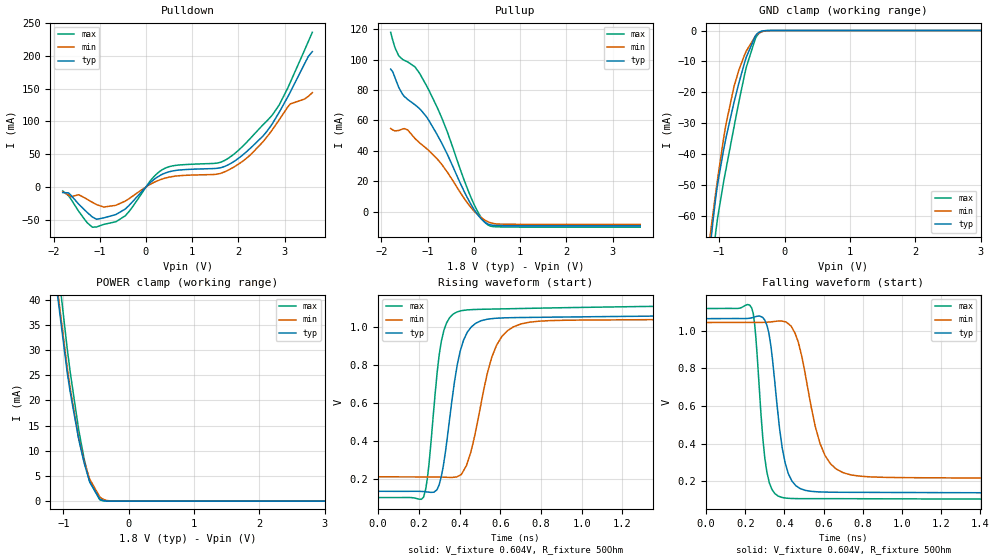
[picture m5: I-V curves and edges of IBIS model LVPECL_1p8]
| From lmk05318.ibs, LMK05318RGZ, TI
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|   LVPECL_1p8 Model
[Model]   LVPECL_1p8
Model_type   3-state
Polarity   Non-Inverting
Vmeas = 0.604
Vref = 0.604
Cref = 2pF
Rref = 50
|   typ   min   max
C_comp   1.5263E-12   1.43105E-12   1.63546E-12
| Where nom  PVT is Nominal Process, 1.8V, 27C
|   Fast PVT is Strong Process,  1.9V, -40C
|   Slow PVT is Weak Process,   1.7V, 125C
[Voltage Range]   1.8   1.7   1.9
|Junction Temperature
[Temperature Range]   27   125   -40
[Pullup Reference]   1.8   1.7   1.9
[Pulldown Reference]   -0   -0   0
[Power Clamp Reference]   1.8   1.7   1.9
[GND Clamp Reference]   0   0   0
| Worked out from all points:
|   slope of the pulldown table from 0 to 0.27 V, typ, clamps not added: 16.8 ohm
|   slope of the pullup table from 0 to 0.27 V, typ, clamps not added: 29.3 ohm
|   GND clamp passes 1 mA (typ) near -0.42 V on its own axis
|   POWER clamp passes 1 mA (typ) near -0.47 V on its own axis
|   falling waveform, V_fixture 0.604V, R_fixture 50Ohm: 20-80 % time 63.4ps typ, 105ps min, 44.6ps max; typ from 1.06 V to 0.136 V
|   rising waveform, V_fixture 0.604V, R_fixture 50Ohm: 20-80 % time 77.1ps typ, 108ps min, 56.9ps max; typ from 0.136 V to 1.06 V
[Pulldown]
|   Voltage   I(typ)   I(min)   I(max)
-1.8V     -8.523mA   -7.443mA   -6.058mA
-1.665V   -9.59mA    -12.82mA   -14.31mA
-1.271V   -38.91mA   -18.85mA   -54.56mA
-1.071V   -49.24mA   -26.78mA   -61.08mA
-444.6mV  -33.56mA   -21.46mA   -43.87mA
106.2mV   7.449mA    4.544mA    10.42mA
408.6mV   21.01mA    13.34mA    28.45mA
1.786V    33.99mA    25.83mA    43.93mA
2.531V    77.56mA    68.77mA    94.79mA
2.887V    114.4mA    102.9mA    125.6mA
3.125V    144.9mA    126.8mA    159.9mA
3.6V      206.5mA    143.9mA    236mA
[GND Clamp]
|   Voltage   I(typ)   I(min)   I(max)
-1.8V     -227.5mA   -244.3mA   -293.8mA
-1.125V   -67.81mA   -64.27mA   -79.09mA
-1.114V   -65.59mA   -62.48mA   -76.82mA
-1.093V   -61.33mA   -58.94mA   -72.53mA
-1.049V   -53.68mA   -52.02mA   -64.8mA
-909mV    -36.18mA   -32mA      -46.42mA
-768.6mV  -22.88mA   -17.82mA   -30.77mA
-585mV    -8.613mA   -6.634mA   -11.87mA
-444.6mV  -1.694mA   -1.777mA   -2.489mA
-385.2mV  -510.7uA   -772.5uA   -830.7uA
-217.8mV  -3.668uA   -26.55uA   -3.583uA
3.6V      0A         0A         0A
[Pullup]
|   Voltage   I(typ)   I(min)   I(max)
-1.8V     93.82mA    54.75mA    118.1mA
-1.708V   88.37mA    53.19mA    108.2mA
-1.627V   81.94mA    53.39mA    102.7mA
-1.433V   73.89mA    53.78mA    98.59mA
-1.265V   70.12mA    47.86mA    94.92mA
-973.8mV  60.02mA    40.15mA    79.97mA
-574.2mV  37.69mA    25.95mA    52.48mA
-72mV     5.208mA    2.981mA    9.959mA
90mV      -2.385mA   -2.254mA   -490uA
262.8mV   -7.547mA   -6.079mA   -7.877mA
522mV     -9.257mA   -8.251mA   -10.13mA
3.6V      -9.435mA   -8.467mA   -10.31mA
[POWER Clamp]
|   Voltage   I(typ)   I(min)   I(max)
-1.8V     167.1mA    290.8mA    175.6mA
-1.103V   42.32mA    43.41mA    48.96mA
-941.4mV  25.56mA    26.6mA     30.29mA
-892.8mV  21.47mA    22.2mA     25.41mA
-774mV    12.9mA     13.11mA    14.91mA
-752.4mV  11.54mA    11.74mA    13.24mA
-682.2mV  7.588mA    7.904mA    8.398mA
-595.8mV  3.783mA    4.344mA    3.83mA
-444.6mV  459.2uA    875.5uA    303.4uA
-352.8mV  57.32uA    198.5uA    23.38uA
-201.6mV  542.8nA    8.178uA    29.43nA
3.6V      0A         0A         0A
[Ramp]
R_load = 50
|   typ   min   max
dV/dt_r   0.557134/7.71003e-11   0.499157/1.08189e-10   0.609207/5.68787e-11
dV/dt_f   0.557302/6.33679e-11   0.498829/1.04825e-10   0.609236/4.4622e-11
[Falling Waveform]
V_fixture = 0.604V
V_fixture_min = 0.632V
V_fixture_max = 0.615V
R_fixture = 50Ohm
C_fixture = 0F
|   Time   V(typ)   V(min)   V(max)
0s        1.065V     1.044V     1.119V
232.8ps   1.069V     1.045V     1.121V
254ps     1.076V     1.045V     964.4mV
299.5ps   1.057V     1.045V     324.4mV
368ps     547.2mV    1.052V     120.5mV
402.7ps   300.3mV    1.048V     110.6mV
457.7ps   176.2mV    977mV      107.3mV
581.4ps   142.7mV    400.8mV    107mV
700.6ps   140.8mV    244.6mV    106.7mV
2.5ns     136mV      212.8mV    103.3mV
[Rising Waveform]
V_fixture = 0.604V
V_fixture_min = 0.632V
V_fixture_max = 0.615V
R_fixture = 50Ohm
C_fixture = 0F
|   Time   V(typ)   V(min)   V(max)
0s        136.2mV    212.3mV    103.3mV
222.7ps   134.9mV    211.9mV    105.1mV
247.5ps   132.1mV    211.9mV    259.1mV
310.2ps   214.8mV    211mV      925.8mV
386.2ps   787.7mV    212mV      1.079V
457.7ps   1.001V     354.4mV    1.092V
536.2ps   1.041V     757.5mV    1.094V
581.4ps   1.046V     904.5mV    1.095V
700.6ps   1.05V      1.016V     1.098V
2.5ns     1.065V     1.044V     1.119V
